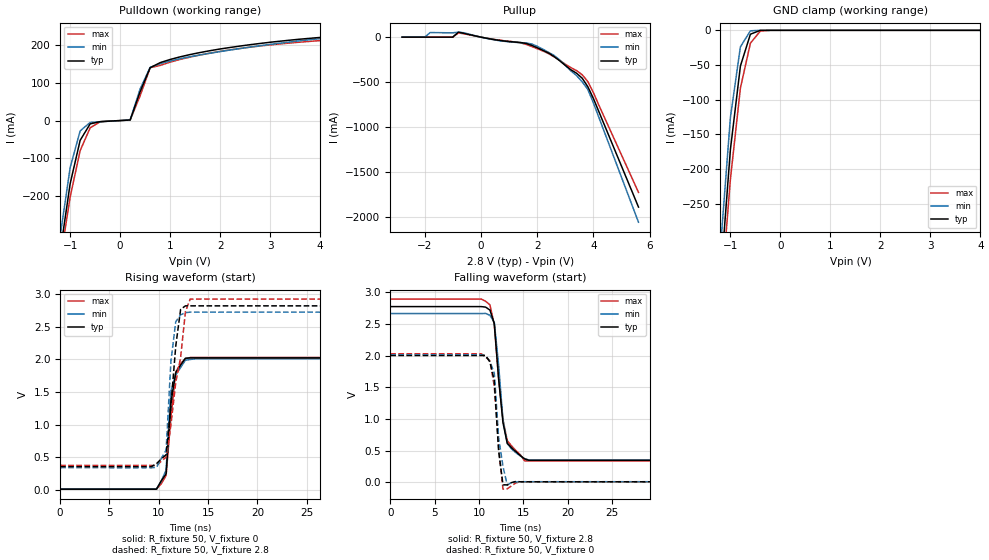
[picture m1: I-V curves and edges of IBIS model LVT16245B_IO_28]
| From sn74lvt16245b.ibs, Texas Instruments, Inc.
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|  Model LVT16245B IO_28
[Model]   LVT16245B_IO_28
Model_type  I/O
Polarity   Non-Inverting
Enable   Active-Low
Vinl = 0.8V
Vinh = 2.0V
Vmeas = 1.5V
Cref = 50pF
Rref = 500
Vref = 0
| variable   typ   min   max
C_comp   10p   NA   NA
[Temperature Range]   40   -25   100
| Ambient Temperature   25   -40   85
[Voltage range]   2.8   2.7   2.9
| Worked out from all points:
|   slope of the pulldown table from 0 to 0.42 V, typ, clamps not added: 5.04 ohm
|   slope of the pullup table from 0 to 0.42 V, typ, clamps not added: 17 ohm
|   GND clamp passes 1 mA (typ) near -0.44 V on its own axis
|   rising waveform, R_fixture 50, V_fixture 0: 20-80 % time 714ps typ, 632ps min, 745ps max; typ from 0.01 V to 2.02 V
|   falling waveform, R_fixture 50, V_fixture 2.8: 20-80 % time 1.02ns typ, 961ps min, 1.13ns max; typ from 2.78 V to 0.35 V
|   rising waveform, R_fixture 50, V_fixture 2.8: 20-80 % time 885ps typ, 636ps min, 1.36ns max; typ from 0.357 V to 2.82 V
|   falling waveform, R_fixture 50, V_fixture 0: 20-80 % time 569ps typ, 756ps min, 722ps max; typ from 2 V to 0.011 V
[Pullup]
|   Voltage   I(typ)   I(min)   I(max)
-2.8V     69.26uA    66.74uA    70.05uA
-2V       67.37uA    64.88uA    67.96uA
-1.8V     66.91uA    50.88mA    67.54uA
-1V       64.06uA    48.11mA    65.69uA
-800mV    56.09mA    54.86mA    46.32mA
600mV     -33.45mA   -36.57mA   -31mA
1.8V      -90.36mA   -75.87mA   -103.1mA
2.6V      -214.8mA   -202.7mA   -218.5mA
3.6V      -456.4mA   -496.7mA   -418.1mA
3.8V      -551.2mA   -581.2mA   -494.3mA
4V        -683.2mA   -732.7mA   -617.6mA
5.6V      -1.888A    -2.056A    -1.725A
[Pulldown]
|   Voltage   I(typ)   I(min)   I(max)
-2.8V     -2.101A    -2.267A    -1.957A
-1.2V     -350.1mA   -307.6mA   -373.4mA
-1V       -167.9mA   -125.1mA   -203.3mA
-800mV    -52.64mA   -27.53mA   -79.93mA
-600mV    -8.881mA   -5.215mA   -19.38mA
-400mV    -2.922mA   -3.265mA   -3.324mA
200mV     1.402mA    1.527mA    1.322mA
400mV     76.88mA    84.05mA    66.06mA
600mV     140.3mA    141.4mA    140.4mA
1V        162.3mA    158.3mA    155.3mA
2V        190.2mA    183.3mA    183.9mA
5.6V      240.8mA    249mA      227.3mA
[GND Clamp]
|   Voltage   I(typ)   I(min)   I(max)
-2.8V     -2.169A    -2.317A    -2.051A
-1.2V     -361.6mA   -314.9mA   -395.8mA
-1V       -171.7mA   -125.6mA   -214.6mA
-800mV    -51.46mA   -23.72mA   -83.26mA
-600mV    -5.57mA    -696.5uA   -18.49mA
-400mV    -29uA      -636nA     -1.001mA
-200mV    -22.97nA   -284.5nA   -3.949uA
5V        67.85nA    1.357uA    140.7nA
[ramp]
| variable   typ   min   max
dV/dt_r   1.200E+00/5.450E-10  1.188E+00/4.880E-10  1.230E+00/5.670E-10
dV/dt_f   1.458E+00/4.580E-10  1.404E+00/3.970E-10  1.518E+00/4.840E-10
R_load = 50
[Rising Waveform]
R_fixture = 50
V_fixture = 0
V_fixture_min = 0
V_fixture_max = 0
C_fixture = 0
L_fixture = 0
|   Time   V(typ)   V(min)   V(max)
0s        10.06mV    10.66mV    10.15mV
9.766ns   10.07mV    12.89mV    10.85mV
10.25ns   138.9mV    131.9mV    93.08mV
10.74ns   244.7mV    304.9mV    219.4mV
11.23ns   1.345V     1.518V     1.118V
11.72ns   1.798V     1.762V     1.807V
12.21ns   1.913V     1.878V     1.938V
12.7ns    2.02V      1.99V      2.01V
13.18ns   2.024V     2V         2.03V
49.71ns   2.024V     2.01V      2.03V
[Falling Waveform]
R_fixture = 50
V_fixture = 2.8
V_fixture_min = 2.7
V_fixture_max = 2.9
C_fixture = 0pf
L_fixture = 0nH
|   Time   V(typ)   V(min)   V(max)
0s        2.777V     2.667V     2.896V
10.25ns   2.777V     2.667V     2.896V
11.23ns   2.722V     2.64V      2.805V
11.72ns   2.509V     2.527V     2.489V
12.21ns   1.638V     1.85V      1.628V
12.7ns    943mV      982.2mV    993.1mV
13.18ns   620.4mV    613.7mV    661.5mV
14.16ns   485.4mV    468.8mV    502.8mV
15.14ns   372.5mV    374.6mV    340.2mV
49.71ns   350.1mV    355.1mV    340.8mV
[Rising Waveform]
R_fixture = 50
V_fixture = 2.8
V_fixture_min = 2.7
V_fixture_max = 2.9
C_fixture = 0pf
L_fixture = 0nH
|   Time   V(typ)   V(min)   V(max)
0s        357mV      339.9mV    375.5mV
9.277ns   357mV      338.8mV    375.5mV
9.766ns   401.4mV    344.5mV    370.4mV
10.74ns   537.6mV    608.4mV    500.8mV
11.23ns   1.297V     1.977V     998.1mV
11.72ns   2.208V     2.581V     1.65V
12.21ns   2.768V     2.685V     2.03V
12.7ns    2.823V     2.719V     2.733V
13.18ns   2.823V     2.726V     2.927V
49.71ns   2.823V     2.726V     2.927V
[Falling Waveform]
R_fixture = 50
V_fixture = 0
V_fixture_min = 0
V_fixture_max = 0
C_fixture = 0pf
L_fixture = 0nH
|   Time   V(typ)   V(min)   V(max)
0s        2.005V     2.018V     2.032V
10.25ns   2.005V     2.018V     2.032V
10.74ns   2.005V     2V         1.98V
11.23ns   1.902V     1.912V     1.921V
11.72ns   1.606V     1.724V     1.521V
12.21ns   495.5mV    707.1mV    550.5mV
12.7ns    -36.58mV   252.8mV    -105.7mV
13.18ns   -38.42mV   -42.8mV    -101mV
14.65ns   10.73mV    11.68mV    11.57mV
49.71ns   10.73mV    11.67mV    11.57mV
